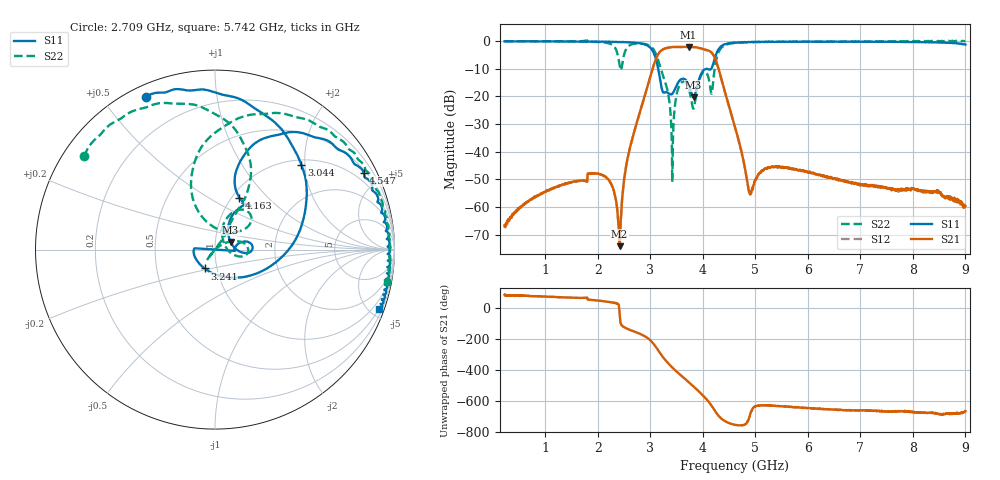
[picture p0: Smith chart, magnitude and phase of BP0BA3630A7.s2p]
!Agilent Technologies,E8358A,US41080443,A.07.50.56
!Agilent E8358A: A.07.50.56
!Date: Friday, December 15, 2017 21:21:56
!Correction: S11(Full 2 Port(1,2))
!S21(Full 2 Port(1,2))
!S12(Full 2 Port(1,2))
!S22(Full 2 Port(1,2))
!S2P File: Measurements: S11, S21, S12, S22:
# Hz S  dB  R 50
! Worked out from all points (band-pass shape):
!   1601 points, 225 MHz to 9 GHz, reference 50 ohm
!   highest |S21| = -2.05 dB at 3.73 GHz (marker M1); lowest = -74.1 dB at 2.413 GHz (marker M2)
!   |S21| within 3 dB of the highest: 3.14 GHz to 4.204 GHz (1.063 GHz wide, 29 % of centre)
!   lowest |S11| = -20.3 dB at 3.823 GHz (marker M3), VSWR 1.21, Z = 59.3 + j5.01 ohm
!   |S11| at or under -10 dB: 3.15 GHz to 4.069 GHz (918.3 MHz wide, 25.4 % of centre); 4.078 GHz to 4.159 GHz (80.69 MHz wide, 1.96 % of centre)
!   |S22| runs from -50.9 to 0.3 dB; largest |S21 - S12| = 0.01
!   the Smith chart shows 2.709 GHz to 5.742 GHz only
!   S11 on the Smith chart (normalised r, x): 2.709 GHz: 0.05, +0.64; 3.044 GHz: 1.11, +1.92; 3.241 GHz: 0.87, -0.19; 4.163 GHz: 1.08, +0.70; 4.547 GHz: 0.62, +4.03; 5.742 GHz: 0.49, -5.71
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2.25e8  -0.05 177.1  -66.61 83.9  -67.35 84.8  0.01 175.9
1.689328e9  -0.13 149.5  -50.30 64.1  -50.36 64.4  0.04 161.3
2.24325e9  -0.26 142.3  -51.30 36.0  -51.36 36.6  -1.05 100.7
2.413266e9  -0.24 135.0  -74.12 -27.4  -72.51 -25.2  -8.49 5.6
2.544891e9  -0.32 127.5  -44.49 -133.3  -44.60 -132.5  -2.66 -174.5
2.709422e9  -0.61 114.5  -31.64 -155.3  -31.72 -155.5  -0.93 144.5
3.043969e9  -3.42 44.4  -9.87 134.4  -10.00 134.5  -2.56 88.5
3.153656e9  -10.32 -20.7  -4.60 83.0  -4.71 83.0  -7.08 63.5
3.241406e9  -18.41 -118.9  -2.94 40.9  -3.03 41.0  -12.42 60.2
3.416906e9  -19.05 5.2  -2.11 -25.3  -2.21 -25.3  -50.91 -132.6
3.548531e9  -14.42 12.9  -2.06 -67.0  -2.16 -66.9  -16.21 15.6
3.729516e9  -15.76 -6.6  -2.05 -119.9  -2.16 -119.9  -17.15 -15.9
3.82275e9  -20.30 25.7  -2.10 -148.3  -2.19 -148.2  -24.37 28.5
4.003734e9  -10.72 57.4  -2.81 153.0  -2.92 153.1  -11.33 55.2
4.162781e9  -9.90 64.8  -4.05 88.8  -4.13 89.0  -18.97 67.3
4.546688e9  -0.61 27.3  -26.63 -31.1  -26.72 -30.6  -0.74 46.0
4.6125e9  -0.50 21.8  -30.98 -37.0  -31.08 -36.5  -0.58 39.4
4.903172e9  -0.37 6.2  -55.15 33.1  -55.45 32.4  -0.37 20.5
5.742281e9  -0.25 -19.7  -46.34 77.2  -46.46 79.1  -0.22 -10.8
6.076828e9  -0.24 -26.5  -47.76 69.7  -47.69 69.1  -0.23 -20.1
7.541156e9  -0.21 -51.7  -53.38 50.3  -53.57 50.0  -0.08 -45.0
9e9  -1.23 -107.4  -59.63 51.9  -60.26 51.9  0.07 -37.1
